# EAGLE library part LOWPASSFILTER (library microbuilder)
Low Pass Filter - RF Signal Filter 0603 869MHz Low Pass Filter - Digikey: 712-1118-1-ND
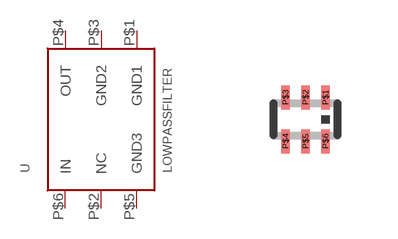
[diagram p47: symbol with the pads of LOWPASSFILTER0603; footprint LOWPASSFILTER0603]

Designator prefix U

## LOWPASSFILTER  [LOWPASSFILTER0603]
P$1  GND1
P$2  NC
P$3  GND2
P$4  OUT
P$5  GND3
P$6  IN

## Footprint LOWPASSFILTER0603 (pad centres in mm)
smd 0.2 x 0.6: P$1 0.5,0.55; P$2 0,0.55; P$3 -0.5,0.55; P$4 -0.5,-0.55; P$5 0,-0.55; P$6 0.5,-0.55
